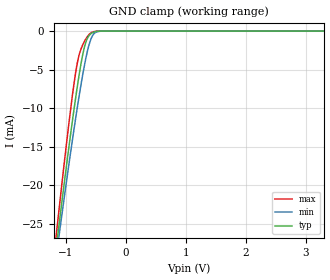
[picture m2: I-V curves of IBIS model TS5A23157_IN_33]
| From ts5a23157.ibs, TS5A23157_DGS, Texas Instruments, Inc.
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[Model]   TS5A23157_IN_33
Model_type  Input
Vinl=1.08
Vinh=2.10
| variable   typ   min   max
C_comp   2.55pF   2.02pF   3.31pF
[Temperature Range]   40   100   -40
| Ambient temperature   25   85   -40
[Voltage range]   3.3   3   3.6
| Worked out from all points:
|   GND clamp passes 1 mA (typ) near -0.64 V on its own axis
[GND Clamp]
| TS5A23157_IN_33
|   Voltage   I(typ)   I(min)   I(max)
-3.3V     -177.8mA   -166mA     -191.8mA
-1.145V   -27.15mA   -28.38mA   -25.39mA
-1.115V   -25.25mA   -26.64mA   -23.27mA
-1.09V    -23.68mA   -25.21mA   -21.51mA
-920mV    -13.37mA   -15.72mA   -10.16mA
-815mV    -7.538mA   -10.24mA   -4.411mA
-765mV    -5.061mA   -7.792mA   -2.746mA
-685mV    -1.948mA   -4.262mA   -1.277mA
-620mV    -671.2uA   -1.985mA   -515.4uA
-560mV    -226.3uA   -672.2uA   -149uA
-375mV    -2.403uA   -5.486uA   -356.1nA
3.3V      76.2pA     212.8pA    43.07pA
